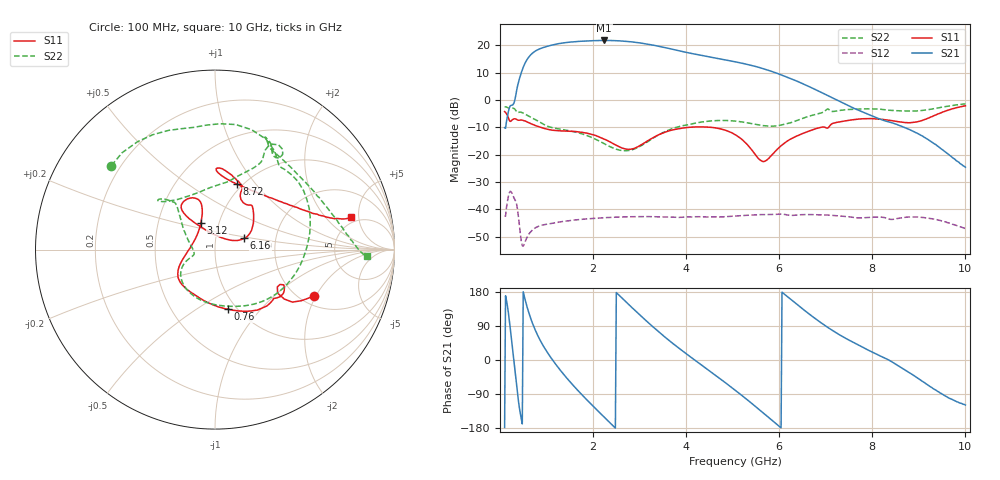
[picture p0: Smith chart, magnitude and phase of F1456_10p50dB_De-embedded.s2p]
! Integrated Device Technology
! Corporate Headquarters
! 6024 Silver Creek Valley Road
! San Jose, CA 95138  USA
! Phone:  1-408-284-8200
! Toll Free:  1-800-223-1366
! Webpage:  http://www.idt.com/
! Timing and RF Division
! 515 Groton Road, Suite 102
! Westford, MA 01886-6024
! Device:  F1456
! Description: 6-bit 0.5 dB Transmit Variable Gain Amplifier
! Frequency:  2100.0 -  2950.00 MHz
! Package:  6x6 mm Thin QFN Plastic Package: 28 pin
! State:  21
! Atten State:  10.5 dB
! Voltage:  +5.00 Volts
! Current:  217.001 mA
! Data:  The device was measured on a the F1455 evaluation board which has
!  individual transmission lines to the RF pins.  Data was collected
!  using a calibrated network analyzer.  The evaluation board was
!  de-embedded using a TRL calibration technique.
!  The reference plane is the edge of the package pin.
!  Pin  1 = CSb
!  Pin  2 = DATA
!  Pin  3 = CLK
!  Pin  4 = RSET
!  Pin  5 = GND
!  Pin  6 = RFIN  = Port 1
!  Pin  7 = GND
!  Pin  8 = NC
!  Pin  9 = NC
!  Pin 10 = NC
!  Pin 11 = NC
!  Pin 12 = NC
!  Pin 13 = NC
!  Pin 14 = /STBY
!  Pin 15 = GND
!  Pin 16 = RFOUT  = Port 2
!  Pin 17 = GND
!  Pin 18 = NC
!  Pin 19 = NC
!  Pin 20 = NC
!  Pin 21 = GND
!  Pin 22 = NC
!  Pin 23 = GND
!  Pin 24 = NC
!  Pin 25 = NC
!  Pin 26 = NC
!  Pin 27 = GND
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# GHz S dB R 50
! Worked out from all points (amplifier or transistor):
!   496 points, 100 MHz to 10 GHz, reference 50 ohm
!   highest |S21| = 21.7 dB at 2.24 GHz (marker M1)
!   |S21| within 3 dB of that: 863.7 MHz to 3.65 GHz (2.787 GHz wide, 123 % of centre)
!   unconditionally stable (mu >= 1): start of sweep to end of sweep
!   at 1.74 GHz: K = 5.77, MAG = 21.9 dB, |S12| = -43.7 dB
!   at 5.06 GHz: K = 10.61, MAG = 14.9 dB, |S12| = -42.4 dB
!   at 10 GHz: K = 212.22, MAG = -15.1 dB, |S12| = -47.0 dB
!   S11 on the Smith chart (normalised r, x): 100 MHz: 2.35, -1.94; 760 MHz: 0.91, -0.68; 3.12 GHz: 0.82, +0.25; 6.16 GHz: 1.37, +0.18; 8.72 GHz: 0.94, +0.81; 10 GHz: 4.34, +3.97
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0.1  -4.29 -25.1  -10.16 -178.0  -42.36 46.2  -2.58 141.0
0.32  -6.89 -32.7  -0.02 -21.3  -36.42 -140.1  -3.38 65.3
0.44  -7.37 -43.2  8.96 -143.1  -49.17 140.8  -4.46 39.2
0.58  -8.01 -59.2  14.67 141.2  -50.26 173.0  -5.62 5.9
0.76  -9.38 -77.5  17.83 78.6  -46.74 131.9  -7.21 -29.5
0.98  -10.54 -98.5  19.38 27.4  -45.49 91.1  -9.29 -66.8
1.2  -11.22 -115.4  20.33 -11.6  -44.87 65.7  -10.41 -95.4
1.5  -11.43 -132.8  21.09 -56.8  -44.06 39.9  -11.30 -125.3
1.76  -11.83 -143.7  21.43 -91.6  -43.61 21.9  -12.39 -142.6
2.24  -14.30 -162.0  21.70 -150.9  -43.04 -6.3  -15.98 -160.1
2.62  -17.56 170.2  21.50 163.7  -42.76 -26.6  -18.52 -168.4
3.12  -15.55 118.1  20.51 106.0  -42.61 -52.3  -15.88 159.9
3.4  -12.81 108.2  19.63 75.6  -42.70 -65.8  -12.89 143.0
4.08  -9.99 114.3  17.07 9.5  -42.75 -95.0  -8.92 131.6
4.6  -10.15 127.1  15.38 -37.6  -42.78 -117.3  -7.60 137.5
5.06  -12.75 130.0  13.89 -80.3  -42.42 -136.9  -7.76 138.9
5.62  -22.29 78.9  11.59 -136.0  -41.91 -166.5  -9.32 123.3
6.16  -15.19 21.1  8.32 168.8  -41.99 160.4  -8.69 84.6
6.7  -11.03 39.9  4.40 116.0  -41.90 131.3  -5.68 63.7
8.36  -7.42 87.1  -8.06 -0.5  -43.54 59.9  -3.78 62.4
8.72  -8.31 71.6  -10.30 -27.4  -42.88 51.0  -4.08 50.3
10  -2.16 13.3  -24.58 -118.8  -46.96 -28.4  -1.46 -2.5
